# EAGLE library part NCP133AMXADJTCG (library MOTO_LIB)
LDO, adjustable output
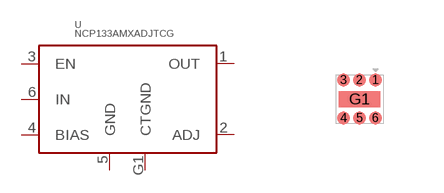
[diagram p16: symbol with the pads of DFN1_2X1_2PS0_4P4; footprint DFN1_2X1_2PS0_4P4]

Designator prefix U

## NCP133AMXADJTCG (MPN: NCP133AMXADJTCG; SUPPLIER: ON SEMI)  [DFN1_2X1_2PS0_4P4]
1  OUT
2  ADJ
3  EN
4  BIAS
5  GND
6  IN
G1  CTGND

## Footprint DFN1_2X1_2PS0_4P4 (pad centres in mm)
smd 0.32 x 0.32: 1 0.4,0.475; 2 0,0.475; 3 -0.4,0.475; 4 -0.4,-0.475; 5 0,-0.475; 6 0.4,-0.475
smd 1.04 x 0.4: G1 0,0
